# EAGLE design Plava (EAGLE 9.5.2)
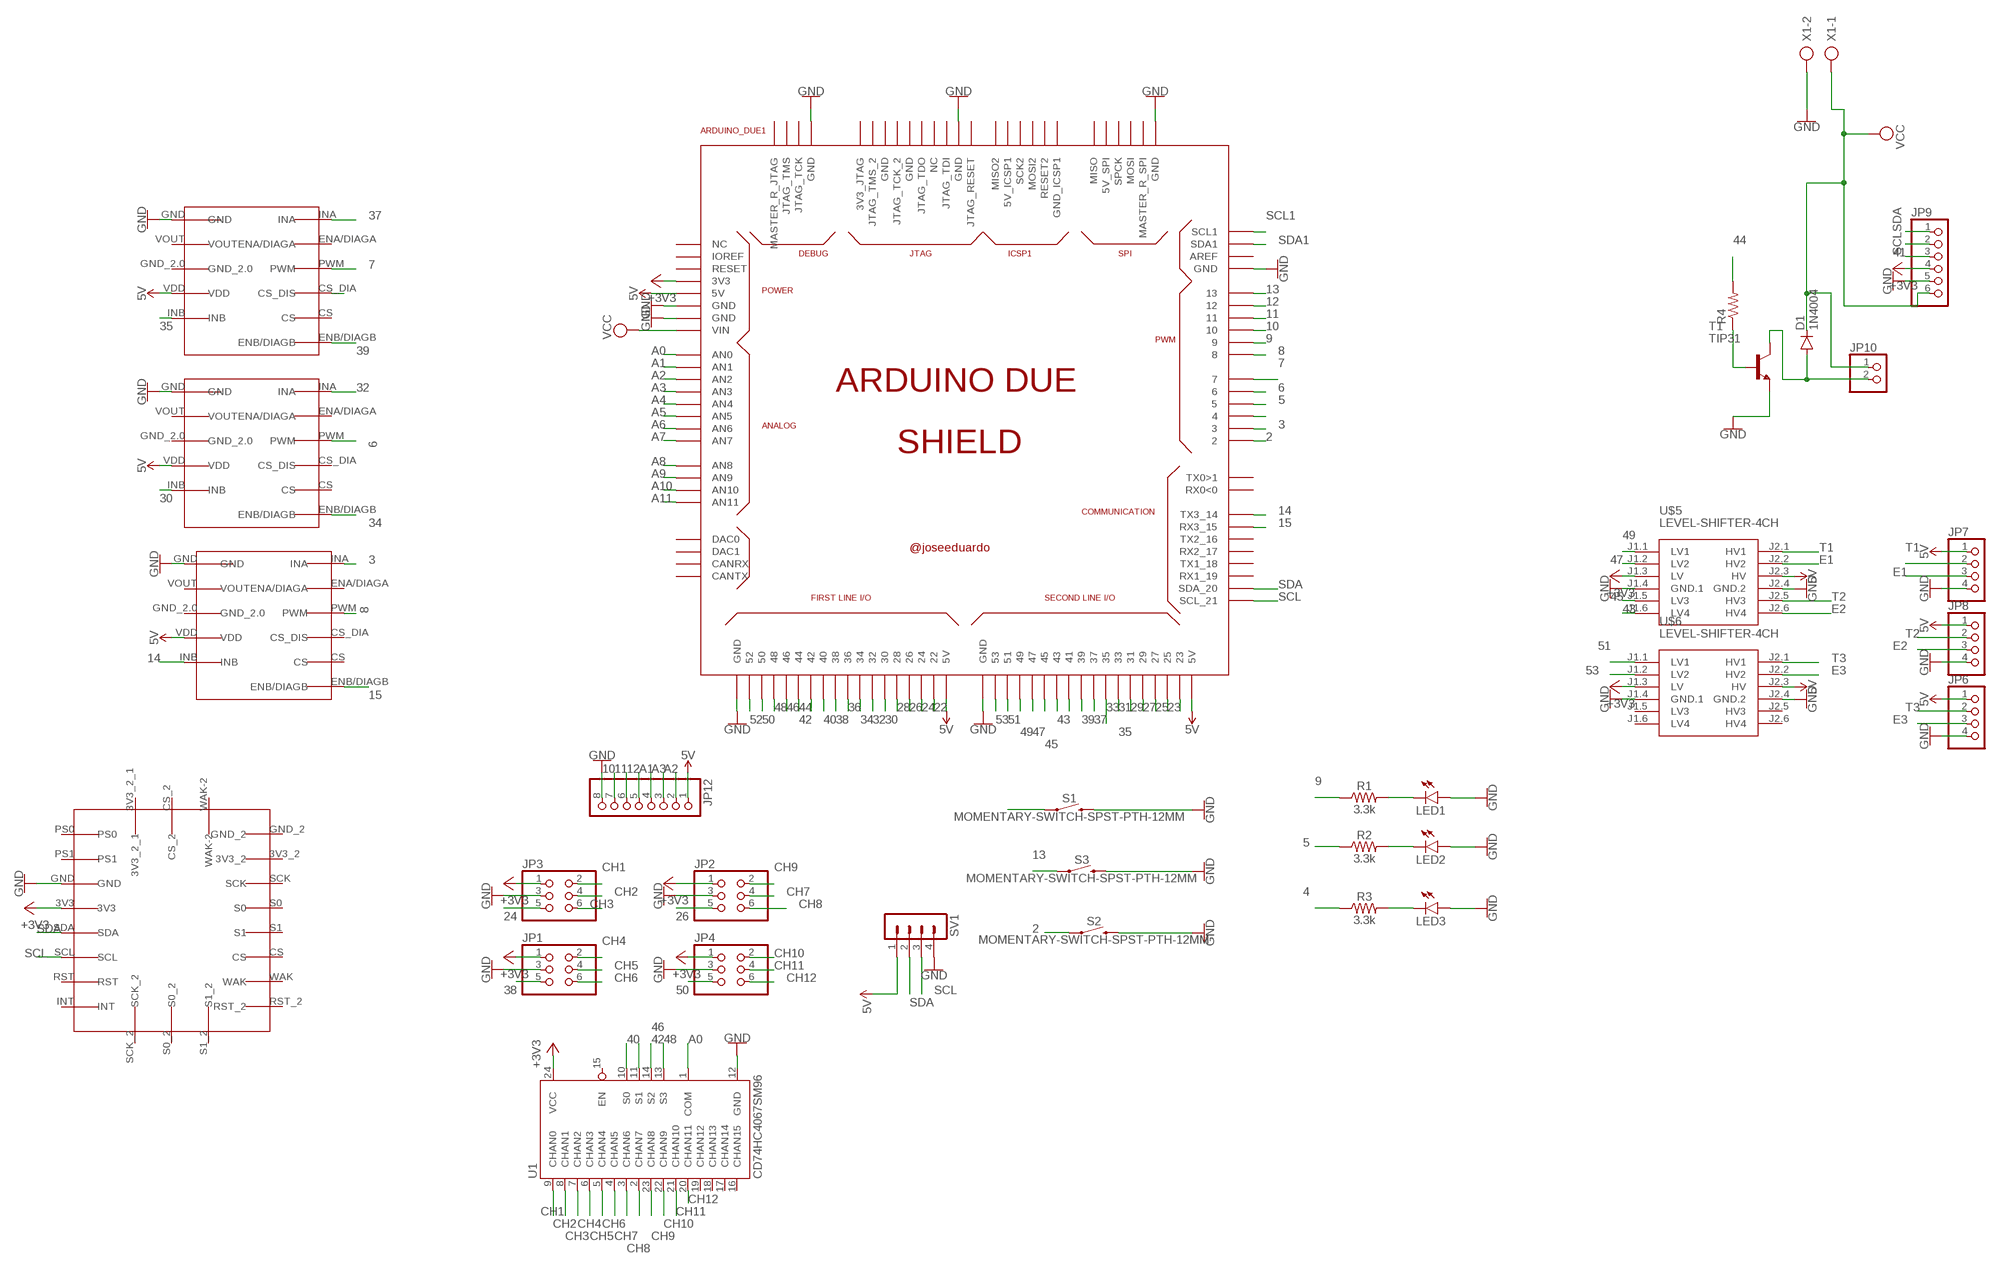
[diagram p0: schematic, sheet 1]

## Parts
ARDUINO_DUE1  ARDUINO_DUE_SHIELD  [ARDUINO_DUE_SHIELD]
D1  1N4004  [DO41-10]
JP1  PINHD-2X3  [2X03]
JP2  PINHD-2X3  [2X03]
JP3  PINHD-2X3  [2X03]
JP4  PINHD-2X3  [2X03]
JP6  PINHD-1X4  [1X04]
JP7  PINHD-1X4  [1X04]
JP8  PINHD-1X4  [1X04]
JP9  PINHD-1X6  [1X06]
JP10  PINHD-1X2  [1X02]
JP12  PINHD-1X8CLEANBIG  [1X08-CLEANBIG]
LED1  LEDCHIP-LED0603  [CHIP-LED0603]
LED2  LEDCHIP-LED0603  [CHIP-LED0603]
LED3  LEDCHIP-LED0603  [CHIP-LED0603]
R1  3.3k  3.3KOHM-0603-1/10W-1%  [0603]
R2  3.3k  3.3KOHM-0603-1/10W-1%  [0603]
R3  3.3k  3.3KOHM-0603-1/10W-1%  [0603]
R4  R-US_0207/7  [0207/7]
S1  MOMENTARY-SWITCH-SPST-PTH-12MM  [TACTILE_SWITCH_PTH_12MM]
S2  MOMENTARY-SWITCH-SPST-PTH-12MM  [TACTILE_SWITCH_PTH_12MM]
S3  MOMENTARY-SWITCH-SPST-PTH-12MM  [TACTILE_SWITCH_PTH_12MM]
SV1  MA04-1  [MA04-1]
T1  TIP31  [TO220]
U1  CD74HC4067SM96  74HC4067SM96  [SSOP24]
U$1  VNH5019_MODULE  [VNH5019]
U$2  VNH5019_MODULE  [VNH5019]
U$3  VNH5019_MODULE  [VNH5019]
U$4  IMU_BNO080  [IMU_BNO080]
U$5  LEVEL-SHIFTER-4CH  [LEVEL-SHIFTER-4CH]
U$6  LEVEL-SHIFTER-4CH  [LEVEL-SHIFTER-4CH]
X1  AK500/2  [AK500/2]

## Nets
2: ARDUINO_DUE1.2 S2.1
3: ARDUINO_DUE1.3 U$3.INA
4: ARDUINO_DUE1.4 R3.1
5: ARDUINO_DUE1.5 R2.1
5V: ARDUINO_DUE1.5V0(5V) ARDUINO_DUE1.5V0_1(5V) ARDUINO_DUE1.5V0_2(5V) JP6.1 JP7.1 JP8.1 JP12.1 SV1.1 U$1.VDD U$2.VDD U$3.VDD U$5.J2.3(HV) U$6.J2.3(HV)
6: ARDUINO_DUE1.6 U$2.PWM
7: ARDUINO_DUE1.7 U$1.PWM
8: ARDUINO_DUE1.8 U$3.PWM
9: ARDUINO_DUE1.9 R1.1
10: ARDUINO_DUE1.10 JP12.7
11: ARDUINO_DUE1.11 JP12.6
12: ARDUINO_DUE1.12 JP12.5
13: ARDUINO_DUE1.13 S3.1
14: ARDUINO_DUE1.14(TX3_14) U$3.INB
15: ARDUINO_DUE1.15(RX3_15) U$3.ENB/DIAGB
22: ARDUINO_DUE1.22
23: ARDUINO_DUE1.23
24: ARDUINO_DUE1.24 JP3.5
25: ARDUINO_DUE1.25
26: ARDUINO_DUE1.26 JP2.5
27: ARDUINO_DUE1.27
28: ARDUINO_DUE1.28
29: ARDUINO_DUE1.29
30: ARDUINO_DUE1.30 U$2.INB
31: ARDUINO_DUE1.31
32: ARDUINO_DUE1.32 U$2.INA
33: ARDUINO_DUE1.33
34: ARDUINO_DUE1.34 U$2.ENB/DIAGB
35: ARDUINO_DUE1.35 U$1.INB
36: ARDUINO_DUE1.36
37: ARDUINO_DUE1.37 U$1.INA
38: ARDUINO_DUE1.38 JP1.5
39: ARDUINO_DUE1.39 U$1.ENB/DIAGB
40: ARDUINO_DUE1.40 U1.10(S0)
41: ARDUINO_DUE1.41 JP9.3
42: ARDUINO_DUE1.42 U1.11(S1)
43: ARDUINO_DUE1.43 U$5.J1.6(LV4)
44: ARDUINO_DUE1.44 R4.2
45: ARDUINO_DUE1.45 U$5.J1.5(LV3)
46: ARDUINO_DUE1.46 U1.14(S2)
47: ARDUINO_DUE1.47 U$5.J1.2(LV2)
48: ARDUINO_DUE1.48 U1.13(S3)
49: ARDUINO_DUE1.49 U$5.J1.1(LV1)
50: ARDUINO_DUE1.50 JP4.5
51: ARDUINO_DUE1.51 U$6.J1.1(LV1)
52: ARDUINO_DUE1.52 S1.1
53: ARDUINO_DUE1.53 U$6.J1.2(LV2)
+3V3: ARDUINO_DUE1.3V3 JP1.1 JP2.1 JP3.1 JP4.1 JP9.4 U1.24(VCC) U$4.3V3 U$5.J1.3(LV) U$6.J1.3(LV)
A0: ARDUINO_DUE1.A0(AN0) U1.1(COM)
A1: ARDUINO_DUE1.A1(AN1) JP12.4
A2: ARDUINO_DUE1.A2(AN2) JP12.2
A3: ARDUINO_DUE1.A3(AN3) JP12.3
A4: ARDUINO_DUE1.A4(AN4)
A5: ARDUINO_DUE1.A5(AN5)
A6: ARDUINO_DUE1.A6(AN6)
A7: ARDUINO_DUE1.A7(AN7)
A8: ARDUINO_DUE1.A8(AN8)
A9: ARDUINO_DUE1.A9(AN9)
A10: ARDUINO_DUE1.A10(AN10)
A11: ARDUINO_DUE1.A11(AN11)
CH1: JP3.2 U1.9(CHAN0)
CH2: JP3.4 U1.8(CHAN1)
CH3: JP3.6 U1.7(CHAN2)
CH4: JP1.2 U1.6(CHAN3)
CH5: JP1.4 U1.5(CHAN4)
CH6: JP1.6 U1.4(CHAN5)
CH7: JP2.4 U1.3(CHAN6)
CH8: JP2.6 U1.2(CHAN7)
CH9: JP2.2 U1.23(CHAN8)
CH10: JP4.2 U1.22(CHAN9)
CH11: JP4.4 U1.21(CHAN10)
CH12: JP4.6 U1.20(CHAN11)
E1: JP7.3 U$5.J2.2(HV2)
E2: JP8.3 U$5.J2.6(HV4)
E3: JP6.3 U$6.J2.2(HV2)
GND: ARDUINO_DUE1.GND ARDUINO_DUE1.GND_1(GND) ARDUINO_DUE1.GND_2(GND) ARDUINO_DUE1.GND_3(GND) ARDUINO_DUE1.GND_4(GND) ARDUINO_DUE1.GND_5(GND) ARDUINO_DUE1.GND_7(GND) ARDUINO_DUE1.GND_10(GND) JP1.3 JP2.3 JP3.3 JP4.3 JP6.4 JP7.4 JP8.4 JP9.5 JP12.8 LED1.A LED2.A LED3.A S1.3 S2.3 S3.3 SV1.4 T1.3(E) U1.12(GND) U$1.GND U$2.GND U$3.GND U$4.GND U$5.J1.4(GND.1) U$5.J2.4(GND.2) U$6.J1.4(GND.1) U$6.J2.4(GND.2) X1.2
N$1: LED1.C R1.2
N$2: LED2.C R2.2
N$3: LED3.C R3.2
N$4: D1.A JP10.2 T1.2(C)
N$5: R4.1 T1.1(B)
N$9: U$1.CS_DIA(CS_DIS)
SCL: ARDUINO_DUE1.21(SCL_21) JP9.2 SV1.3 U$4.SCL
SCL1: ARDUINO_DUE1.SCL1
SDA: ARDUINO_DUE1.20(SDA_20) JP9.1 SV1.2 U$4.SDA
SDA1: ARDUINO_DUE1.SDA1
T1: JP7.2 U$5.J2.1(HV1)
T2: JP8.2 U$5.J2.5(HV3)
T3: JP6.2 U$6.J2.1(HV1)
VCC: ARDUINO_DUE1.VIN D1.C JP9.6 JP10.1 X1.1
Unconnected: ARDUINO_DUE1.0(RX0<0) ARDUINO_DUE1.1(TX0>1) ARDUINO_DUE1.3V3_JTAG ARDUINO_DUE1.5V_2(5V_SPI) ARDUINO_DUE1.5V_ICSP1 ARDUINO_DUE1.16(TX2_16) ARDUINO_DUE1.17(RX2_17) ARDUINO_DUE1.18(TX1_18) ARDUINO_DUE1.19(RX1_19) ARDUINO_DUE1.AREF ARDUINO_DUE1.CANRX ARDUINO_DUE1.CANTX ARDUINO_DUE1.DAC0 ARDUINO_DUE1.DAC1 ARDUINO_DUE1.GND_8(GND) ARDUINO_DUE1.GND_9(GND) ARDUINO_DUE1.GND_ICSP1 ARDUINO_DUE1.IOREF ARDUINO_DUE1.JTAG_RESET ARDUINO_DUE1.JTAG_TCK ARDUINO_DUE1.JTAG_TCK_2 ARDUINO_DUE1.JTAG_TDI ARDUINO_DUE1.JTAG_TDO ARDUINO_DUE1.JTAG_TMS ARDUINO_DUE1.JTAG_TMS_2 ARDUINO_DUE1.MASTER_RESET_JTAG(MASTER_R_JTAG) ARDUINO_DUE1.MASTER_RESET_SPI(MASTER_R_SPI) ARDUINO_DUE1.MISO ARDUINO_DUE1.MISO2 ARDUINO_DUE1.MOSI ARDUINO_DUE1.MOSI2 ARDUINO_DUE1.NC_2(NC) ARDUINO_DUE1.NC_5(NC) ARDUINO_DUE1.RESET ARDUINO_DUE1.RESET2 ARDUINO_DUE1.SCK2 ARDUINO_DUE1.SPCK U1.15(EN) U1.16(CHAN15) U1.17(CHAN14) U1.18(CHAN13) U1.19(CHAN12) U$1.CS U$1.ENA/DIAGA U$1.GND_2.0 U$1.VOUT U$2.CS U$2.CS_DIA(CS_DIS) U$2.ENA/DIAGA U$2.GND_2.0 U$2.VOUT U$3.CS U$3.CS_DIA(CS_DIS) U$3.ENA/DIAGA U$3.GND_2.0 U$3.VOUT U$4.3V3_2 U$4.3V3_2_1 U$4.CS U$4.CS_2 U$4.GND_2 U$4.INT U$4.PS0 U$4.PS1 U$4.RST U$4.RST_2 U$4.S0 U$4.S0_2 U$4.S1 U$4.S1_2 U$4.SCK U$4.SCK_2 U$4.WAK U$4.WAK-2 U$6.J1.5(LV3) U$6.J1.6(LV4) U$6.J2.5(HV3) U$6.J2.6(HV4)

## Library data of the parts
ARDUINO_DUE1 = arduino_due_shield:ARDUINO_DUE_SHIELD
D1 = diode:1N4004: DIODE
JP1-JP4 = pinhead:PINHD-2X3: PIN HEADER
JP6-JP8 = pinhead:PINHD-1X4: PIN HEADER
JP9 = adafruit:PINHD-1X6: PIN HEADER
JP10 = pinhead:PINHD-1X2: PIN HEADER
JP12 = adafruit:PINHD-1X8: PIN HEADER
LED1-LED3 = led:LED: LED
R1-R3 = SparkFun-Resistors:3.3KOHM: 3.3kΩ resistor; PROD_ID: RES-07851
R4 = rcl:R-US_: RESISTOR, American symbol; SPICEPREFIX: R
S1-S3 = SparkFun-Switches:MOMENTARY-SWITCH-SPST: Momentary Switch (Pushbutton) - SPST; PROD_ID: SWCH-09185; SF_SKU: COM-09190
SV1 = con-lstb:MA04-1: PIN HEADER; OC_FARNELL: unknown; OC_NEWARK: unknown
T1 = transistor:TIP31: NPN Transistor Medium Power Linear Switching Applications Source: http://onsemi.com
U1 = SparkFun-IC-Logic:74*4067: 16-channel analog MUX Datasheet SparkFun Products MP3 Trigger (WIG-13720) SparkFun Analog/Digital MUX Breakout - CD74HC4067 (BOB-09056); PROD_ID: IC-08252
U$1-U$3 = Puente_h_mamalon:VNH5019_MODULE
U$4 = IMU bno080:IMU_BNO080
U$5 U$6 = diy-modules:LEVEL-SHIFTER-4CH: 4-Channel Bi-Directional Logic Level Converter based on BSS128 transistors Click here to find device on ebay.com
X1 = con-ptr500:AK500/2: CONNECTOR; OC_FARNELL: unknown; OC_NEWARK: unknown

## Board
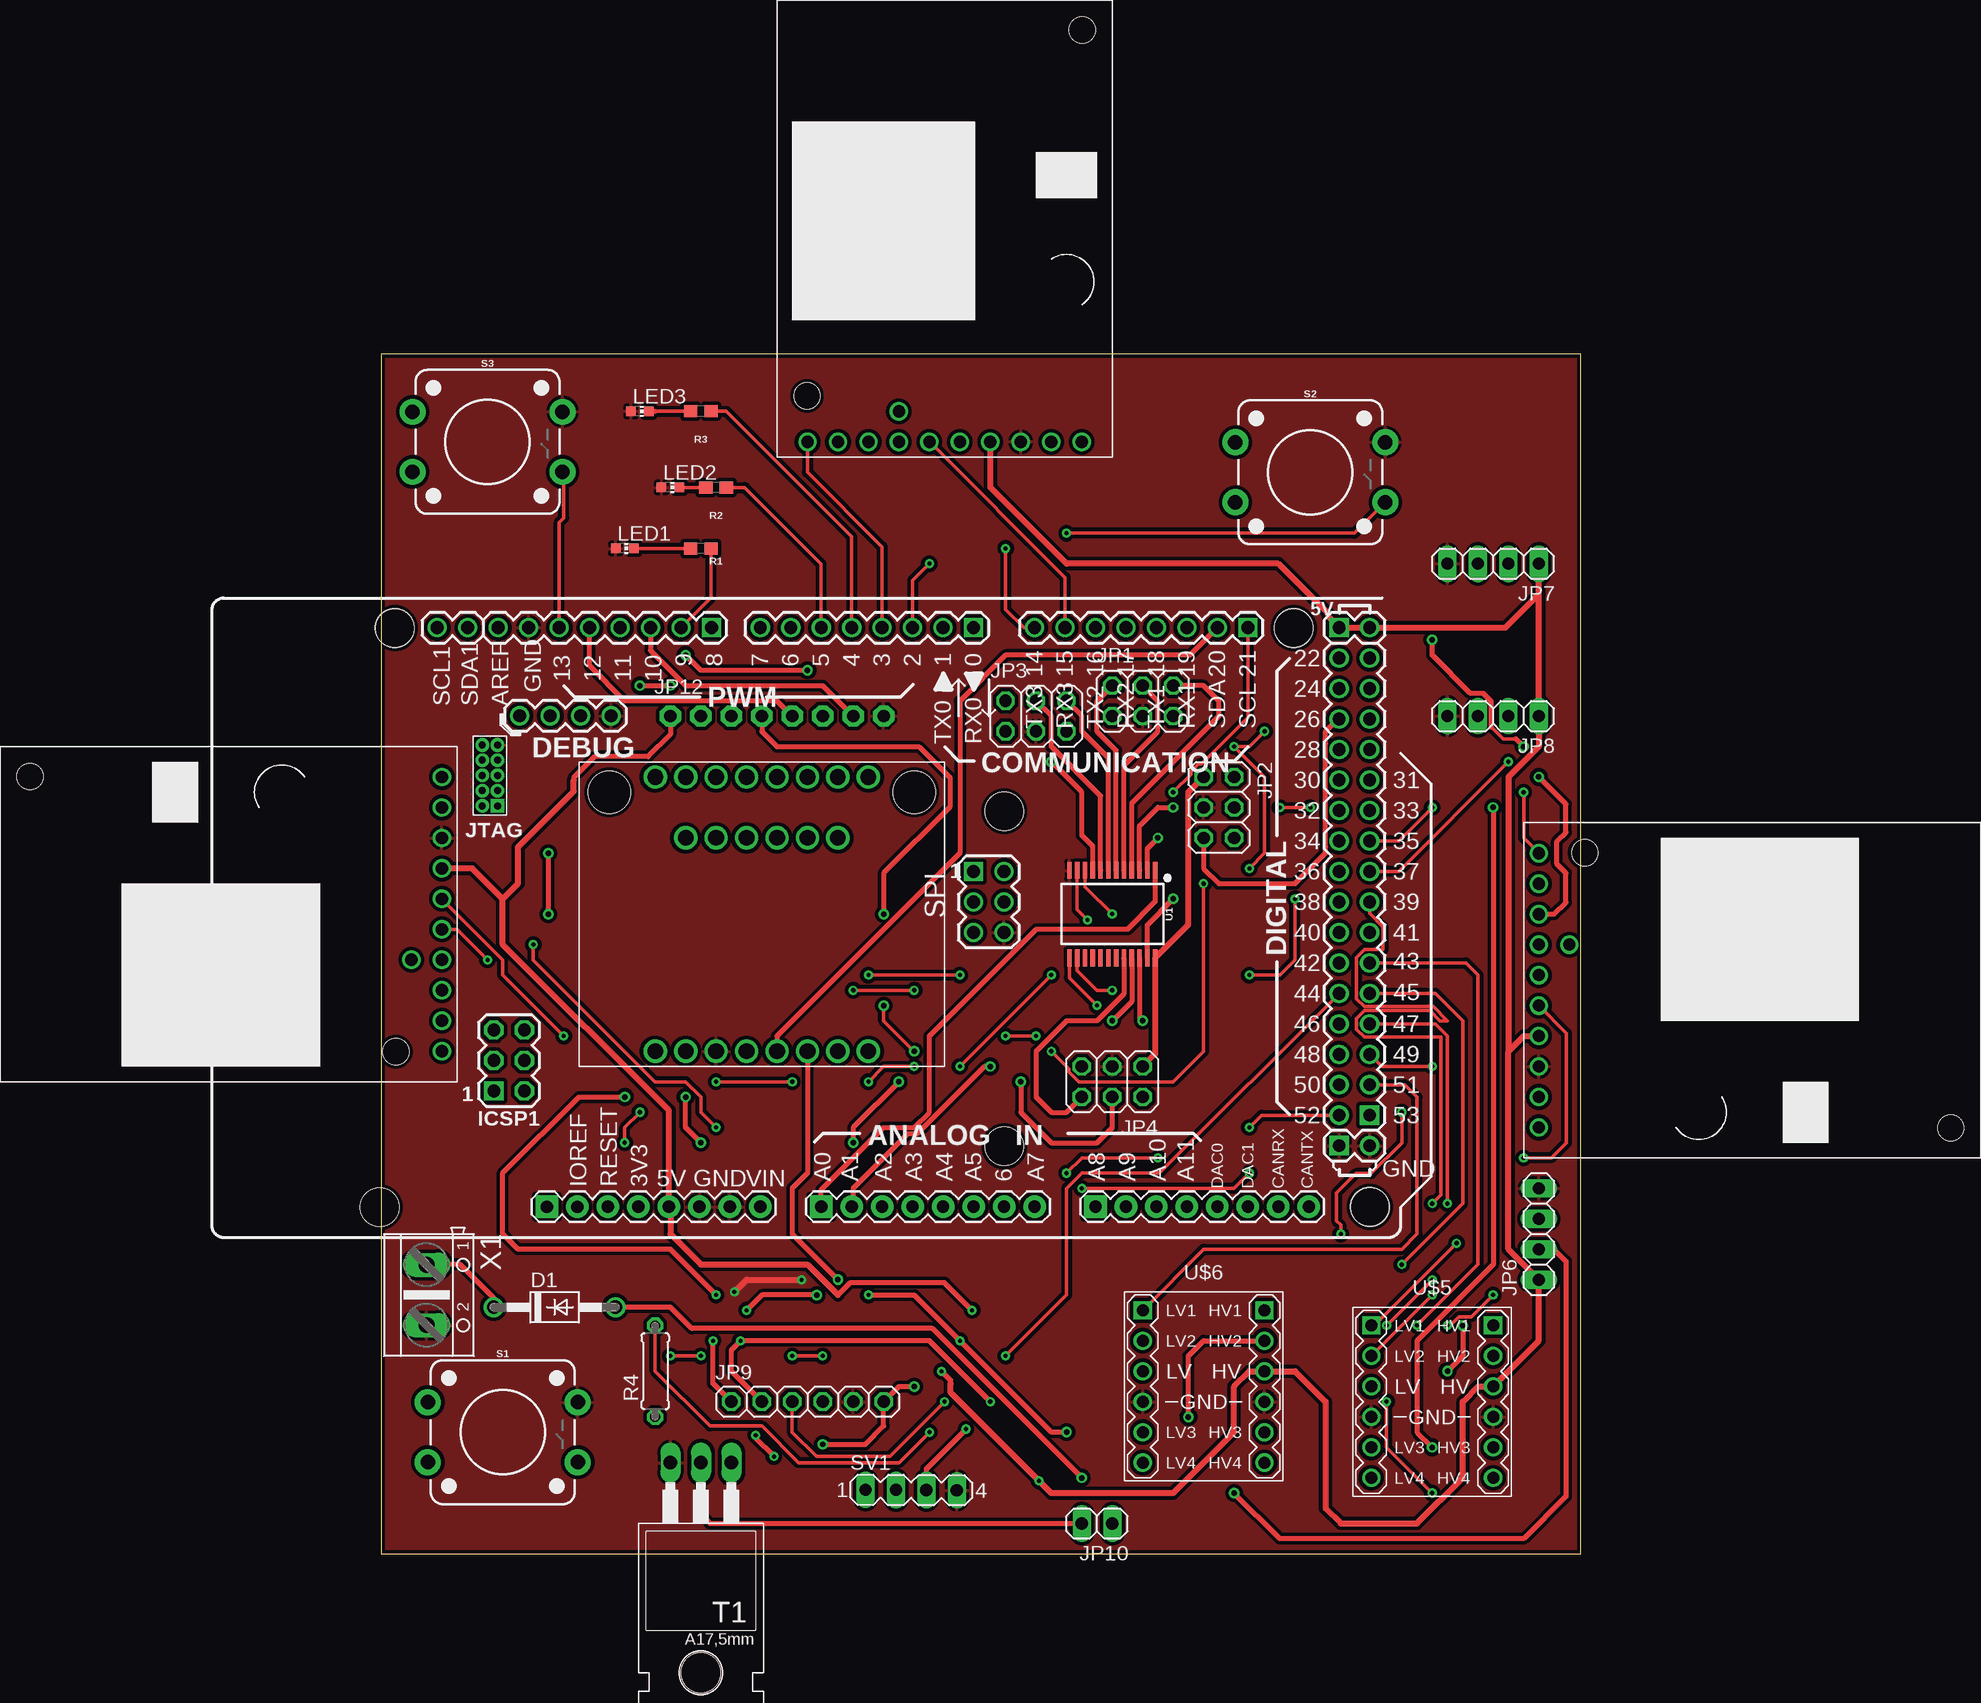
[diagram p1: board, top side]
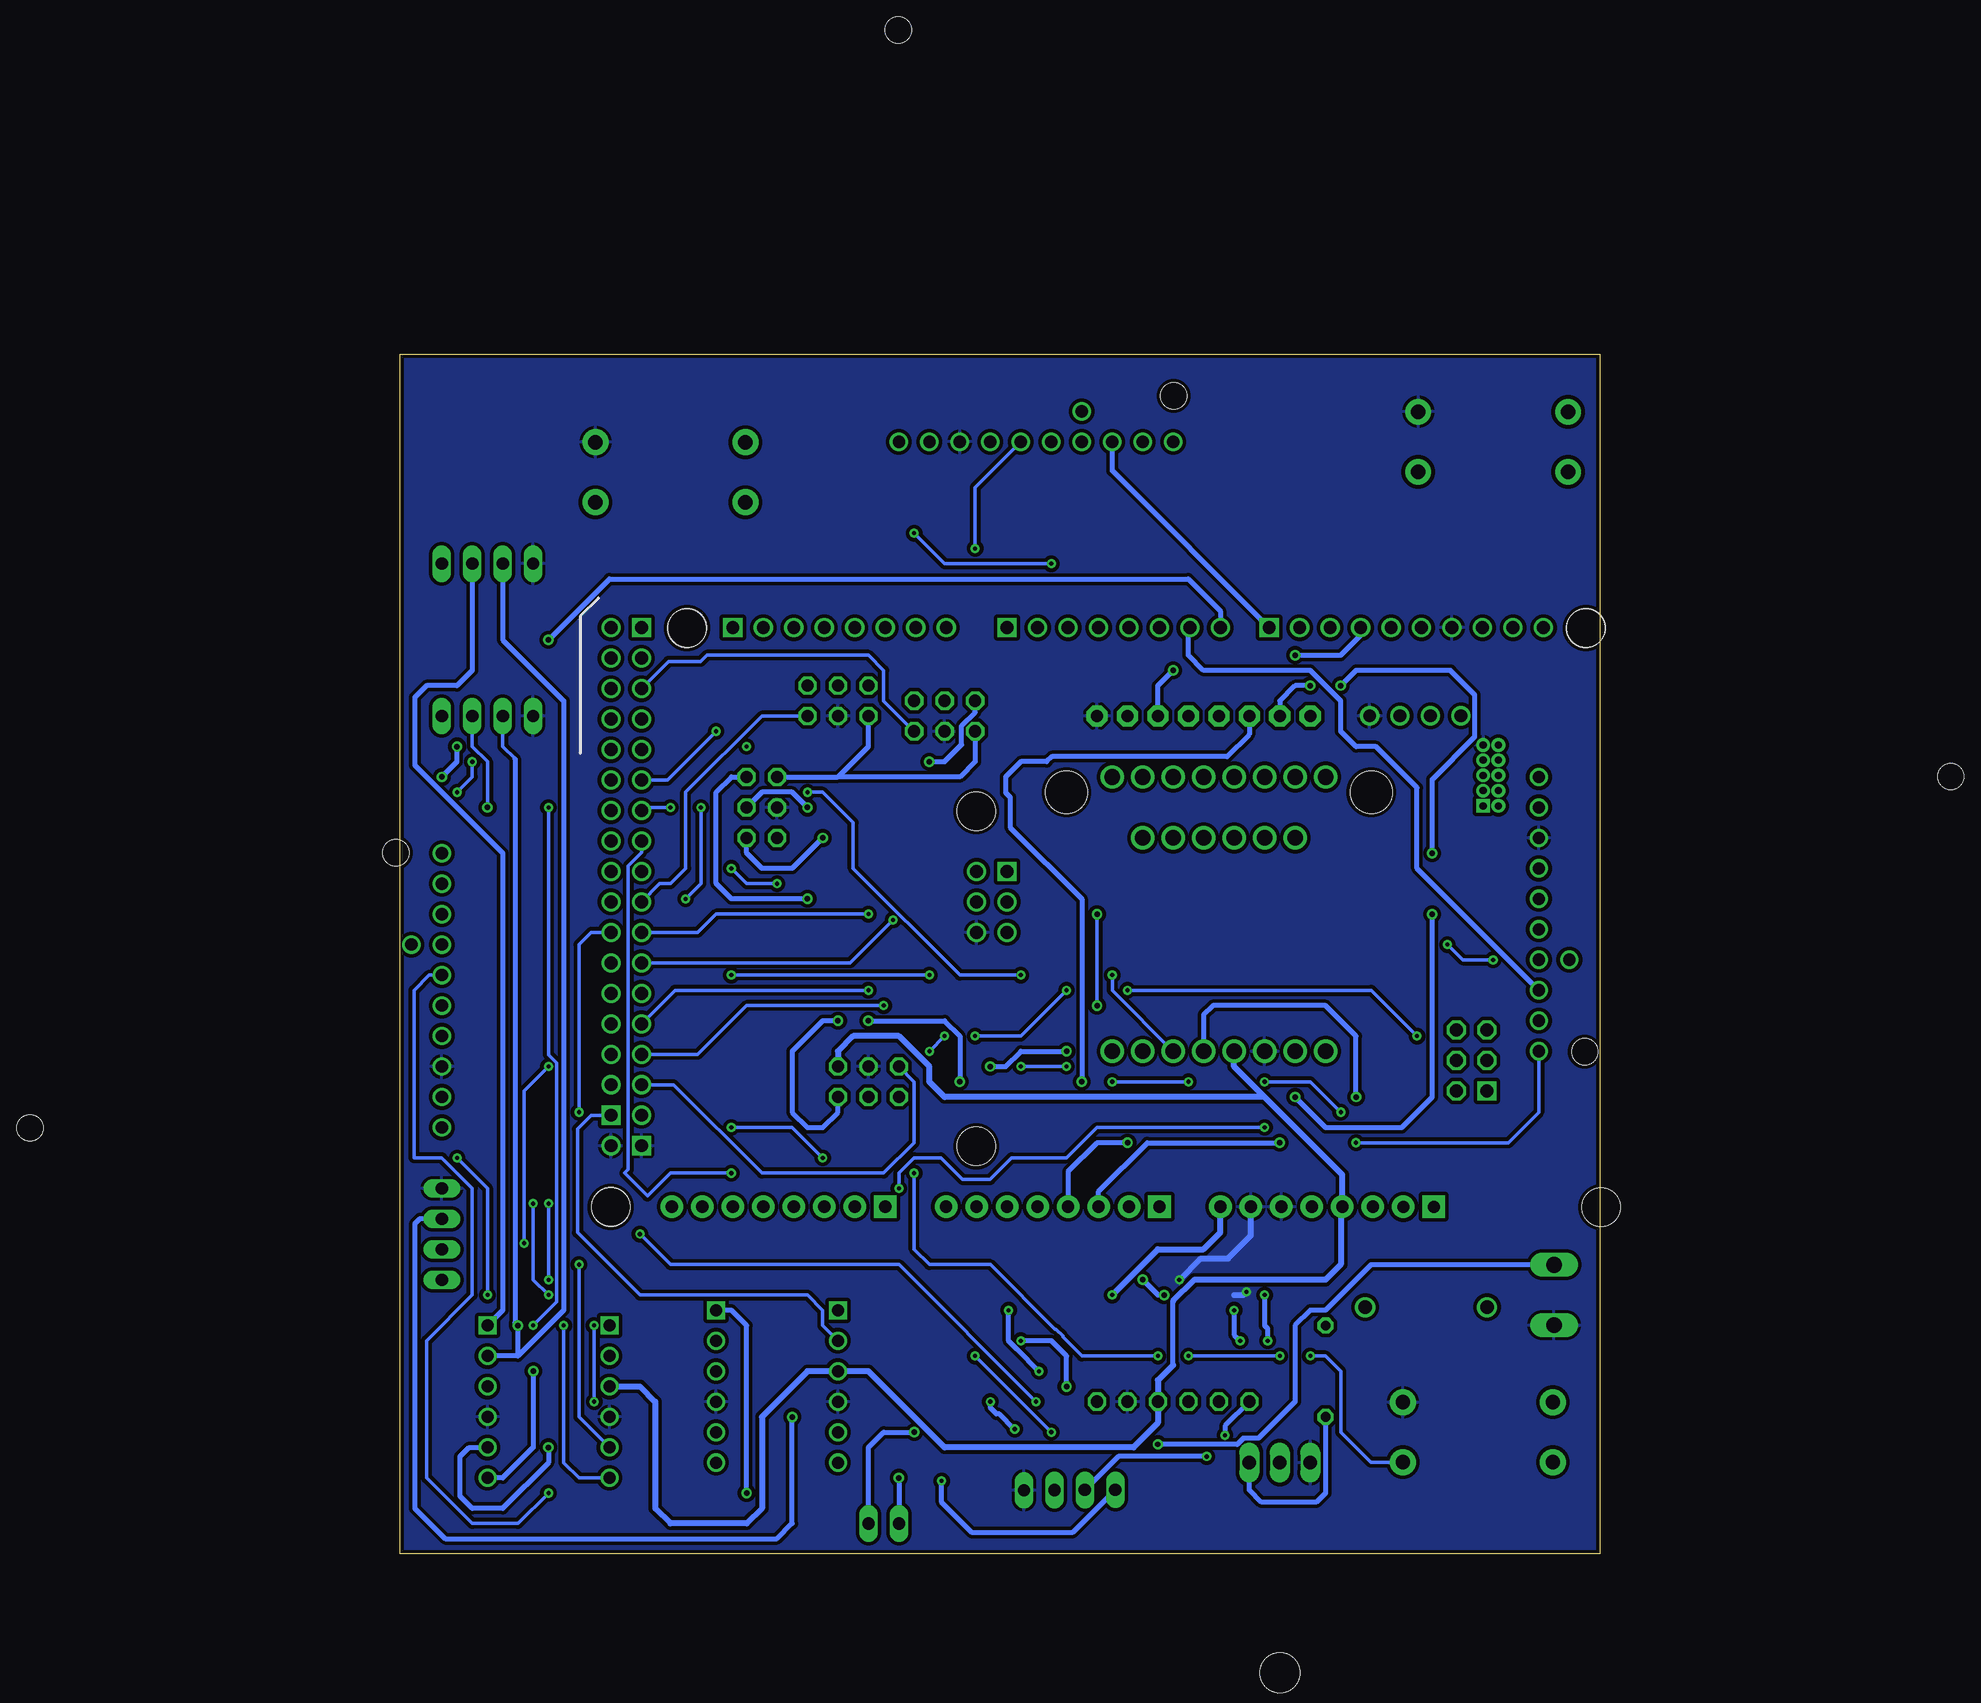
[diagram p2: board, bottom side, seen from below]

Size 100 x 100 mm. Coordinates in mm from the lower left corner, seen from the top.
Outline: 0,0 100,0 100,100 0,100 0,0
Copper layers (1*16): Top 0.035mm / dielectric 1.5mm / Bottom 0.035mm
Design rules "default *": minimum track width 6mil, minimum drill 0.35mm, track to track 6mil, track to pad 6mil, pad to pad 6mil, via to via 6mil, smd to smd 6mil, copper to edge 10mil, drill to drill 6mil, minimum pad ring 10mil, minimum via ring 8mil, stop-mask expansion 4mil, vias tented up to drill 0mil, thermal gap 10mil

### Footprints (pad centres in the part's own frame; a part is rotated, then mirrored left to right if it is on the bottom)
ARDUINO_DUE_SHIELD = drill 1.067 square: 0 63.373,51.816; 5V0_1 93.853,51.816; 8 41.529,51.816; 21 86.233,51.816; 53 96.393,11.176; GND_2 93.853,8.636; MISO 63.373,31.496; MISO2 23.384,13.196 | drill 1.067: 1 60.833,51.816; 2 58.293,51.816; 3 55.753,51.816; 4 53.213,51.816; 5 50.673,51.816; 5V0_2 96.393,51.816; 5V_2 65.913,31.496; 6 48.133,51.816; 7 45.593,51.816; 9 38.989,51.816; 10 36.449,51.816; 11 33.909,51.816; 12 31.369,51.816; 13 28.829,51.816; 14 68.453,51.816; 15 70.993,51.816; 16 73.533,51.816; 17 76.073,51.816; 18 78.613,51.816; 19 81.153,51.816; 20 83.693,51.816; 22 93.853,49.276; 23 96.393,49.276; 24 93.853,46.736; 25 96.393,46.736; 26 93.853,44.196; 27 96.393,44.196; 28 93.853,41.656; 29 96.393,41.656; 30 93.853,39.116; 31 96.393,39.116; 32 93.853,36.576; 33 96.393,36.576; 34 93.853,34.036; 35 96.393,34.036; 36 93.853,31.496; 37 96.393,31.496; 38 93.853,28.956; 39 96.393,28.956; 40 93.853,26.416; 41 96.393,26.416; 42 93.853,23.876; 43 96.393,23.876; 44 93.853,21.336; 45 96.393,21.336; 46 93.853,18.796; 47 96.393,18.796; 48 93.853,16.256; 49 96.393,16.256; 50 93.853,13.716; 51 96.393,13.716; 52 93.853,11.176; AREF 23.749,51.816; GND_3 96.393,8.636; GND_4 26.289,51.816; GND_5 65.913,26.416; GND_7 33.161,44.473; JTAG_TCK 30.621,44.473; JTAG_TMS 28.081,44.473; MASTER_RESET_JTAG 25.541,44.473; MASTER_RESET_SPI 63.373,26.416; MOSI 65.913,28.956; SCL1 18.669,51.816; SDA1 21.209,51.816; SPCK 63.373,28.956 | drill 1.016 pad 1.88: 3V3 35.433,3.556; 5V0 37.973,3.556; A1 53.213,3.556; A2 55.753,3.556; A3 58.293,3.556; A4 60.833,3.556; A5 63.373,3.556; A6 65.913,3.556; A7 68.453,3.556; A9 76.073,3.556; A10 78.613,3.556; A11 81.153,3.556; CANRX 88.773,3.556; CANTX 91.313,3.556; DAC0 83.693,3.556; DAC1 86.233,3.556; GND 40.513,3.556; GND_1 43.053,3.556; IOREF 30.346,3.543; RESET 32.893,3.555; VIN 45.593,3.556 | drill 0.6 pad 1.016 square: 3V3_JTAG 23.689,36.964 | drill 1.067 octagon: 5V_ICSP1 25.924,13.196; GND_ICSP1 25.924,18.276; MOSI2 25.924,15.736; RESET2 23.384,18.276; SCK2 23.384,15.736 | drill 1.016 pad 1.88 square: A0 50.673,3.556; A8 73.533,3.556; NC_2 27.806,3.543 | drill 0.6 pad 1.143: GND_8 23.689,38.234; GND_9 23.689,40.774; GND_10 23.689,42.044; JTAG_RESET 22.419,42.044; JTAG_TCK_2 22.419,38.234; JTAG_TDI 22.419,40.774; JTAG_TDO 22.419,39.504; JTAG_TMS_2 22.419,36.964; NC_5 23.689,39.504 | hole 3.2: 15.113,51.816; 90.043,51.816; 96.393,3.556; 96.418,3.505; 15.138,51.765; 90.068,51.765; 13.868,3.505; 65.938,36.525; 65.938,8.585
DO41-10 = drill 1.118: A 5.08,0; C -5.08,0
2X03 = drill 1.016 octagon: 1 -2.54,-1.27; 2 -2.54,1.27; 3 0,-1.27; 4 0,1.27; 5 2.54,-1.27; 6 2.54,1.27
1X04 = drill 1.016 long: 1 -3.81,0; 2 -1.27,0; 3 1.27,0; 4 3.81,0
1X06 = drill 1.016 octagon: 1 -6.35,0; 2 -3.81,0; 3 -1.27,0; 4 1.27,0; 5 3.81,0; 6 6.35,0
1X02 = drill 1.016 long: 1 -1.27,0; 2 1.27,0
1X08-CLEANBIG = drill 1.016 pad 1.778 octagon: 1 -8.89,0; 2 -6.35,0; 3 -3.81,0; 4 -1.27,0; 5 1.27,0; 6 3.81,0; 7 6.35,0; 8 8.89,0
CHIP-LED0603 = smd 0.8 x 0.8: A 0,-0.75; C 0,0.75
0603 = smd 1.1 x 1: 1 -0.85,0; 2 0.85,0
0207/7 = drill 0.813 octagon: 1 -3.81,0; 2 3.81,0
TACTILE_SWITCH_PTH_12MM = drill 1.2 pad 2.159: 1 6.25,-2.5; 2 -6.25,-2.5; 3 6.25,2.5; 4 -6.25,2.5
MA04-1 = drill 1.016 long: 1 -3.81,0; 2 -1.27,0; 3 1.27,0; 4 3.81,0
TO220 = drill 1.118 long: 1 -2.54,-6.35; 2 0,-6.35; 3 2.54,-6.35 | hole 3.302: 0,11.176
SSOP24 = smd 0.348 x 1.397: 1 -3.575,-3.656; 2 -2.925,-3.656; 3 -2.275,-3.656; 4 -1.625,-3.656; 5 -0.975,-3.656; 6 -0.325,-3.656; 7 0.325,-3.656; 8 0.975,-3.656; 9 1.625,-3.656; 10 2.275,-3.656; 11 2.925,-3.656; 12 3.575,-3.656; 13 3.575,3.656; 14 2.925,3.656; 15 2.275,3.656; 16 1.625,3.656; 17 0.975,3.656; 18 0.325,3.656; 19 -0.325,3.656; 20 -0.975,3.656; 21 -1.625,3.656; 22 -2.275,3.656; 23 -2.925,3.656; 24 -3.575,3.656
VNH5019 = drill 1.02: CS 10.16,1.27; CS_DIA 10.16,3.81; ENA/DIAGA 5.08,1.27; ENB/DIAGB 12.7,1.27; GND 20.32,1.27; GND_2.0 25.4,1.27; INA 2.54,1.27; INB 15.24,1.27; PWM 7.62,1.27; VDD 17.78,1.27; VOUT 22.86,1.27 | hole 2.18: 2.5,5.1; 25.44,35.6
IMU_BNO080 = drill 1.3: 3V3 13.97,1.27; 3V3_2 8.89,24.13; 3V3_2_1 8.89,19.05; CS 19.05,24.13; CS_2 19.05,19.05; GND 11.43,1.27; GND_2 6.35,24.13; INT 24.13,1.27; PS0 6.35,1.27; PS1 8.89,1.27; RST 21.59,1.27; RST_2 24.13,24.13; S0 13.97,24.13; S0_2 13.97,19.05; S1 16.51,24.13; S1_2 16.51,19.05; SCK 11.43,24.13; SCK_2 11.43,19.05; SCL 19.05,1.27; SDA 16.51,1.27; WAK 21.59,24.13; WAK-2 21.59,19.05 | hole 3.5: 2.54,22.86; 27.94,22.86
LEVEL-SHIFTER-4CH = drill 1 square: J1.1 -5.08,6.35; J2.1 5.08,6.35 | drill 1: J1.2 -5.08,3.81; J1.3 -5.08,1.27; J1.4 -5.08,-1.27; J1.5 -5.08,-3.81; J1.6 -5.08,-6.35; J2.2 5.08,3.81; J2.3 5.08,1.27; J2.4 5.08,-1.27; J2.5 5.08,-3.81; J2.6 5.08,-6.35
AK500/2 = drill 1.321 long: 1 -2.515,0; 2 2.515,0

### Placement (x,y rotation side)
ARDUINO_DUE1  -13.97,25.4 0 top
D1  14.48,20.57 0 top
JP1  63.5,71.12 0 top
JP2  69.85,62.23 270 top
JP3  54.61,69.85 0 top
JP4  60.96,39.37 180 top
JP6  96.52,26.67 90 top
JP7  92.71,82.55 180 top
JP8  92.71,69.85 180 top
JP9  35.56,12.7 0 top
JP10  59.69,2.54 180 top
JP12  33.02,69.85 0 top
LED1  20.32,83.82 270 top
LED2  24.13,88.9 270 top
LED3  21.59,95.25 270 top
R1  26.67,83.82 180 top
R2  27.94,88.9 180 top
R3  26.67,95.25 180 top
R4  22.86,15.24 90 top
S1  10.16,10.16 0 top
S2  77.47,90.17 0 top
S3  8.89,92.71 0 top
SV1  44.2,5.33 359.7 top
T1  26.67,1.27 180 top
U1  60.96,53.34 180 top
U$1  95.25,60.96 270 top
U$2  6.35,39.37 90 top
U$3  33.02,91.44 0 top
U$4  16.51,40.64 0 top
U$5  87.63,12.7 0 top
U$6  68.58,13.97 0 top
X1  3.81,21.59 270 top

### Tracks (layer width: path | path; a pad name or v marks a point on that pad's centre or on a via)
2  (via drill 0.35)
  Top 0.305: S2.1 81.14,85.09 v57.15,85.09 | v45.72,82.55 44.32,81.15 ARDUINO_DUE1.2
  Bottom 0.305: v57.15,85.09 54.61,82.55 v45.72,82.55
3
  Top 0.305: U$3.INA 35.56,90.17 41.78,83.95 ARDUINO_DUE1.3
4
  Top 0.305: R3.1 28.79,95.25 39.24,84.8 ARDUINO_DUE1.4
5
  Top 0.305: R2.1 30.31,88.9 36.7,82.51 ARDUINO_DUE1.5
5V  (via drill 0.35)
  Top 0.406: JP12.1 24.13,68.33 22.27,66.47 17.82,66.47 16.08,64.73 16.08,64.52 | 47.5,14.22 47.5,14.48 v46.74,15.24 | v49.28,20.32 46.99,22.61 39.12,22.61 38.1,21.59
  Top 0.508: 38.1,21.59 35.56,24.13 26.67,24.13 24.13,26.67 24.13,28.83 ARDUINO_DUE1.5V0 24,36.96 10.16,50.8 10.16,54.61 | 96.52,80.01 93.73,77.22 ARDUINO_DUE1.5V0_2 ARDUINO_DUE1.5V0_1 78.97,78.13 78.97,78.38 74.8,82.55 57.15,82.55 50.8,88.9 U$3.VDD | 96.52,80.01 JP7.1 | 96.52,80.01 JP8.1 96.52,67.31 93.98,64.77 93.98,41.91 | 10.16,54.61 7.62,57.15 U$2.VDD | 93.98,41.91 95.25,43.18 U$1.VDD | 93.98,41.91 93.98,25.4 JP6.1 96.52,17.78 U$5.J2.3 91.44,13.97 90.17,12.7 90.17,6.35 86.36,2.54 80.01,2.54 78.74,3.81 78.74,12.7 76.2,15.24 U$6.J2.3 72.39,15.24 71.12,13.97 71.12,10.16 66.04,5.08 55.88,5.08 v54.86,6.1 47.5,13.46 47.5,14.22 | 10.16,54.61 11.43,55.88 11.43,58.93 16.08,63.58 16.08,64.52
  Bottom 0.406: SV1.1 43.96,1.78 52.32,1.78 54.86,4.32 v54.86,6.1 | v46.74,15.24 48.54,17.05 48.56,17.05 49.28,17.76 v49.28,20.32
6
  Bottom 0.406: U$2.PWM 15.24,57.15 15.24,63.89 18.66,67.31 20.32,67.31 21.59,68.58 21.59,71.12 24.13,73.66 33.02,73.66 34.29,74.93 34.29,77.09 ARDUINO_DUE1.6
7  (via drill 0.46)
  Top 0.305: 94.61,67.94 93.54,67.94 92.56,68.93
  Top 0.406: U$1.PWM 97.79,53.34 98.78,54.33 98.78,56.76 98.04,57.5 98.04,59.42 98.78,60.16 98.78,62.51 v96.52,64.77 | v87.63,76.2 87.63,74.93 90.83,71.73 91.9,71.73 92.56,71.08 92.56,68.93 | v95.25,67.31 94.61,67.94 94.59,67.97
  Bottom 0.406: v96.52,64.77 95.25,66.04 v95.25,67.31 | v87.63,76.2 82.55,81.28 34.29,81.28 31.62,78.61 ARDUINO_DUE1.7
8
  Bottom 0.406: ARDUINO_DUE1.8 40.64,90.3 U$3.PWM
9
  Top 0.305: ARDUINO_DUE1.9 27.52,79.72 R1.1
10
  Top 0.406: ARDUINO_DUE1.10 22.48,75.31 25.4,72.39 36.83,72.39 JP12.7
11  (via drill 0.46)
  Top 0.406: v35.56,73.66 26.67,73.66 v25.4,74.93
  Bottom 0.406: JP12.6 36.83,72.39 v35.56,73.66 | v25.4,74.93 21.59,74.93 19.94,76.58 ARDUINO_DUE1.11
12
  Top 0.406: JP12.5 33.02,71.12 20.32,71.12 17.4,74.04 ARDUINO_DUE1.12
13
  Top 0.305: ARDUINO_DUE1.13 14.86,85.98 15.24,86.36 15.24,90.11 S3.1
14  (via drill 0.35)
  Top 0.305: v52.07,83.82 52.07,78.74 53.59,77.22 ARDUINO_DUE1.14
  Bottom 0.305: U$3.INB 52.07,88.9 v52.07,83.82
15
  Top 0.305: U$3.ENB/DIAGB 57.02,81.41 ARDUINO_DUE1.15
24
  Bottom 0.305: ARDUINO_DUE1.24 77.62,74.4 74.95,74.4 74.42,74.93 60.96,74.93 59.69,73.66 59.69,71.12 JP3.5
26
  Top 0.406: JP2.5 68.58,57.15 69.85,55.88 76.2,55.88 78.74,58.42 78.74,58.95 78.73,58.96 78.73,67.53 78.74,67.55 78.74,68.58 79.76,69.6 ARDUINO_DUE1.26
30  (via drill 0.35)
  Top 0.305: v73.66,68.58 72.39,67.31 v71.12,67.31 73.66,64.77 73.66,58.42 v72.39,57.15 | v68.58,55.88 68.58,41.91 66.04,39.37 58.18,39.37 57.35,40.2 57.35,40.44 v55.88,41.91 | v54.61,43.18 v52.07,43.18 | v44.45,46.99 v39.37,46.99 | v15.24,43.18 10.16,48.26 10.16,49.53 U$2.INB
  Bottom 0.305: ARDUINO_DUE1.30 77.72,64.52 v73.66,68.58 | v72.39,57.15 71.12,55.88 v68.58,55.88 | v55.88,41.91 v54.61,43.18 | v52.07,43.18 48.26,43.18 v44.45,46.99 | v39.37,46.99 19.05,46.99 v15.24,43.18
32  (via drill 0.35)
  Top 0.305: v20.32,34.29 20.32,35.56 v21.59,36.83 | v27.94,39.37 v34.29,39.37 | v40.64,39.37 41.91,40.64 v44.45,40.64 | v48.26,40.64 v55.88,48.26 | v72.39,48.26 74.93,48.26 76.2,49.53 v76.2,54.61 | v74.93,62.23 v77.47,62.23
  Bottom 0.305: U$2.INA 5.08,36.83 7.62,34.29 v20.32,34.29 | v21.59,36.83 24.13,39.37 v27.94,39.37 | v34.29,39.37 v40.64,39.37 | v44.45,40.64 v48.26,40.64 | v55.88,48.26 v72.39,48.26 | v76.2,54.61 74.93,55.88 v74.93,62.23 | v77.47,62.23 79.63,62.23 ARDUINO_DUE1.32
34  (via drill 0.35)
  Top 0.305: v72.39,31.75 71.12,30.48 v58.42,30.48 | v27.94,35.56 26.67,36.83 26.67,38.1 25.4,39.37 22.86,39.37 12.7,49.53 v12.7,50.8 | v8.89,49.53 6.35,52.07 U$2.ENB/DIAGB
  Bottom 0.305: ARDUINO_DUE1.34 79.88,58.46 80.99,57.35 80.99,32.04 81.28,31.75 79.38,29.84 77.47,31.75 v72.39,31.75 | v58.42,30.48 58.42,31.75 57.15,33.02 54.92,33.02 53.12,31.22 50.82,31.22 49.02,33.02 44.45,33.02 41.91,35.56 v27.94,35.56 | v12.7,50.8 11.43,49.53 v8.89,49.53
35  (via drill 0.35)
  Top 0.305: U$1.INB 98.83,43.41 98.83,34.29 97.56,33.02 v95.25,33.02 | v92.71,21.59 90.91,19.79 89.86,19.79 89.13,19.05 v88.9,19.05 | v87.63,62.23 84.84,59.44 ARDUINO_DUE1.35
  Bottom 0.305: v95.25,33.02 92.71,30.48 v92.71,21.59 | v87.63,62.23 87.63,41.61 86.95,40.92 86.95,21 v88.9,19.05
37  (via drill 0.35)
  Top 0.305: U$1.INA 95.25,59.69 v95.25,63.5 | v93.98,66.04 84.84,56.9 ARDUINO_DUE1.37
  Bottom 0.305: v95.25,63.5 93.98,64.77 v93.98,66.04
38
  Bottom 0.305: JP1.5 69.85,69.85 76.2,63.5 76.2,57.15 77.47,55.88 78.36,55.88 ARDUINO_DUE1.38
39  (via drill 0.35)
  Top 0.305: ARDUINO_DUE1.39 82.42,53.38 83.53,52.27 83.53,50.38 81.97,50.38 81.32,49.73 81.32,46.28 81.97,45.63 87.72,45.63 88.9,44.45 88.28,44.45 87.43,45.3 81.97,45.3 81.32,44.65 81.32,43.74 81.97,43.09 88.34,43.09 88.34,29.92 v87.63,29.21 | v87.63,22.86 83.83,19.07 v83.83,19.05 | v83.82,12.7 83.82,8.89 v87.63,5.08
  Bottom 0.305: v87.63,29.21 v87.63,22.86 | v83.83,19.05 83.83,12.71 v83.82,12.7 | v87.63,5.08 90.17,2.54 93.98,2.54 97.79,6.35 97.79,17.78 93.98,21.59 93.98,30.48 96.52,33.02 98.83,33.02 98.83,46.99 97.56,48.26 U$1.ENB/DIAGB
40  (via drill 0.35)
  Top 0.305: U1.10 58.69,55.62 v60.96,53.34
  Bottom 0.305: v60.96,53.34 73.66,53.34 75.18,51.82 ARDUINO_DUE1.40
41  (via drill 0.35)
  Top 0.305: JP9.3 34.29,10.16 36.3,8.15 42.44,8.15 v46.99,12.7 | v85.09,36.83 85.09,34.29 82.53,31.73 81.28,31.73 79.65,30.1 79.65,27.78 80.01,27.43 v80.01,26.67
  Bottom 0.305: ARDUINO_DUE1.41 84.07,51.82 85.09,50.8 v85.09,36.83 | v80.01,26.67 77.47,24.13 58.42,24.13 v46.99,12.7
42  (via drill 0.35)
  Top 0.305: U1.11 58.03,53.73 v58.9,52.86
  Bottom 0.305: v58.9,52.86 62.48,49.28 ARDUINO_DUE1.42
43  (via drill 0.35)
  Top 0.305: ARDUINO_DUE1.43 90.42,49.28 91.44,48.26 91.44,24.13 v86.36,19.05
  Bottom 0.305: v86.36,19.05 86.36,7.62 85.09,6.35 U$5.J1.6
44  (via drill 0.35)
  Top 0.305: ARDUINO_DUE1.44 64.9,31.75 58.42,31.75 57.15,30.48 57.15,21.59 v52.07,16.51 | v45.72,10.16 43.18,7.62 34.8,7.62 31.75,10.67 27.43,10.67 22.86,15.24 R4.2
  Bottom 0.305: v52.07,16.51 v45.72,10.16
45  (via drill 0.35)
  Top 0.305: v85.09,24.13 90.17,29.21 90.17,44.45 87.88,46.74 ARDUINO_DUE1.45
  Bottom 0.305: U$5.J1.5 85.09,11.43 v85.09,24.13
46  (via drill 0.35)
  Top 0.305: U1.14 58.03,48.65 59.69,46.99 v60.96,46.99
  Bottom 0.305: v60.96,46.99 77.09,46.99 ARDUINO_DUE1.46
47  (via drill 0.35)
  Top 0.305: ARDUINO_DUE1.47 87.88,44.2 88.9,43.18 v88.9,29.21 | v87.63,21.59 U$5.J1.2
  Bottom 0.305: v88.9,29.21 88.9,22.86 v87.63,21.59
48  (via drill 0.35)
  Top 0.305: U1.13 57.38,48.02 v59.69,45.72
  Bottom 0.305: v59.69,45.72 71.12,45.72 75.18,41.66 ARDUINO_DUE1.48
49  (via drill 0.35)
  Top 0.305: v89.66,25.91 82.8,19.05 U$5.J1.1 | v87.63,40.64 83.44,40.64 ARDUINO_DUE1.49
  Bottom 0.305: v89.66,25.91 89.66,38.61 v87.63,40.64
50
  Bottom 0.305: JP4.5 57.15,39.37 57.15,34.29 59.69,31.75 69.85,31.75 77.22,39.12 ARDUINO_DUE1.50
51
  Top 0.305: U$6.J1.1 68.58,25.4 85.09,25.4 86.36,26.67 86.36,38.1 85.34,39.12 ARDUINO_DUE1.51
52  (via drill 0.35)
  Top 0.305: v24.13,16.51 v26.67,16.51 | v34.29,16.51 v36.83,16.51 | v57.15,31.75 58.42,33.02 v64.77,33.02 | v72.39,35.56 73.41,36.58 ARDUINO_DUE1.52
  Bottom 0.305: S1.1 19.09,7.66 21.59,10.16 21.59,15.24 22.86,16.51 v24.13,16.51 | v26.67,16.51 v34.29,16.51 | v36.83,16.51 43.18,16.51 44.76,18.09 44.76,18.18 45.32,18.74 45.41,18.74 50.8,24.13 55.88,24.13 57.15,25.4 v57.15,31.75 | v64.77,33.02 67.31,35.56 v72.39,35.56
53
  Bottom 0.305: ARDUINO_DUE1.53 84.07,36.58 85.22,35.43 85.22,26.8 80.01,21.59 66.04,21.59 64.77,20.32 64.77,19.05 U$6.J1.2
+3V3
  Top 0.508: JP4.1 64.53,41.67 U1.24 67.31,52.46 67.31,63.5 JP2.1
  Bottom 0.406: JP2.1 63.5,64.77 | JP1.1 60.96,67.31 63.5,64.77 | JP3.1 52.07,66.04 53.34,64.77 63.5,64.77 | 35.56,15.75 35.56,21.08
  Bottom 0.508: U$4.3V3 30.48,40.64 27.94,38.1 | 27.94,38.1 21.46,31.62 ARDUINO_DUE1.3V3 21.59,28.83 21.59,24.13 22.86,22.86 33.78,22.86 35.56,21.08 | 35.56,15.75 36.83,14.48 JP9.4 36.83,10.92 38.86,8.89 54.61,8.89 60.96,15.24 U$6.J1.3 66.04,15.24 69.85,11.43 69.85,3.81 71.12,2.54 77.47,2.54 78.74,3.81 78.74,12.7 80.01,13.97 U$5.J1.3 | 27.94,38.1 54.61,38.1 55.88,39.37 55.88,40.64 58.42,43.18 62.23,43.18 63.5,41.91 JP4.1
A0
  Top 0.406: U1.1 64.53,54.38 62.23,52.07 54.61,52.07 45.72,43.18 45.72,36.83 44.45,35.56 41.91,35.56 36.7,30.35 ARDUINO_DUE1.A0
A1  (via drill 0.46)
  Top 0.305: v44.45,41.91 41.91,44.45 v41.91,45.72
  Top 0.406: JP12.4 31.75,68.58 33.02,67.31 44.84,67.31 47.42,64.73 47.42,62.27 41.91,56.76 v41.91,53.34 | v50.8,40.64 50.32,40.64 44.68,35 43.89,35 39.37,30.48 39.37,29.08 ARDUINO_DUE1.A1
  Bottom 0.305: v41.91,53.34 v41.91,45.72
  Bottom 0.406: v50.8,40.64 49.53,40.64 48.26,41.91 v44.45,41.91
A2  (via drill 0.46)
  Top 0.406: v26.67,34.29 25.4,35.56 v25.4,38.1 | v13.97,53.34 v13.97,58.42 | v21.59,72.39 v24.13,72.39
  Bottom 0.406: ARDUINO_DUE1.A2 41.78,30.23 37.72,34.29 v26.67,34.29 | v25.4,38.1 22.86,35.56 16.51,35.56 13.97,38.1 v13.97,53.34 | v13.97,58.42 13.97,64.57 10.41,68.12 10.41,71.62 12.45,73.66 20.32,73.66 v21.59,72.39 | JP12.2 26.67,71.12 25.4,72.39 v24.13,72.39
A3  (via drill 0.46)
  Top 0.406: v43.18,39.37 39.37,35.56 v39.37,34.29
  Bottom 0.406: JP12.3 29.21,68.33 31.07,66.47 45.68,66.47 46.11,66.04 48.26,66.04 49.53,64.77 49.53,63.47 49.15,63.09 49.15,60.58 43.18,54.61 v43.18,39.37 | v39.37,34.29 41.91,34.29 44.32,31.88 ARDUINO_DUE1.A3
CH1  (via drill 0.46)
  Top 0.406: v55.88,66.04 58.42,63.5 58.42,59.91 59.34,58.99 U1.9
  Bottom 0.406: v55.88,66.04 54.61,66.04 53.19,67.46 53.19,69.04 52.07,70.16 JP3.2
CH2
  Top 0.406: U1.8 59.98,63.2 55.88,67.31 55.88,69.85 JP3.4
CH3
  Top 0.406: U1.7 60.63,66.36 58.42,68.58 58.42,69.85 JP3.6
CH4
  Top 0.406: U1.6 61.28,66.98 59.69,68.58 59.69,71.12 JP1.2
CH5
  Top 0.406: U1.5 61.94,65.75 64.77,68.58 64.77,71.12 JP1.4
CH6
  Top 0.406: U1.4 62.59,62.59 69.85,69.85 69.85,71.12 68.58,72.39 JP1.6
CH7  (via drill 0.46)
  Top 0.406: U1.3 63.23,60.7 64.77,62.23 v66.04,62.23
  Bottom 0.406: v66.04,62.23 67.31,63.5 69.85,63.5 JP2.4
CH8  (via drill 0.46)
  Top 0.406: U1.2 63.88,58.8 v64.77,59.69
  Bottom 0.406: v64.77,59.69 67.31,57.15 69.85,57.15 71.12,58.42 JP2.6
CH9  (via drill 0.46)
  Top 0.406: U1.23 63.88,52.45 v66.04,54.61
  Bottom 0.406: v66.04,54.61 72.39,54.61 73.66,55.88 73.66,63.5 72.39,64.77 JP2.2
CH10  (via drill 0.46)
  Top 0.406: U1.22 63.23,44.72 v63.5,44.45
  Bottom 0.406: v63.5,44.45 64.77,44.45 67.31,41.91 67.31,36.83 66.04,35.56 64.77,35.56 63.5,36.83 JP4.2
CH11  (via drill 0.46)
  Top 0.406: U1.21 62.59,46.08 v60.96,44.45 | v53.34,39.37 53.34,36.83 55.88,34.29 59.69,34.29 60.96,35.56 JP4.4
  Bottom 0.406: v60.96,44.45 54.61,44.45 53.34,43.18 v53.34,39.37
CH12
  Top 0.406: U1.20 61.94,46.7 59.69,44.45 57.15,44.45 54.61,41.91 54.61,38.1 55.88,36.83 57.15,36.83 JP4.6
E1
  Bottom 0.406: JP7.3 91.44,76.2 86.36,71.12 86.36,20.32 90.17,16.51 U$5.J2.2
E2  (via drill 0.46)
  Top 0.406: v90.17,19.05 90.17,16.51 v88.9,15.24
  Bottom 0.305: JP8.3 91.44,67.31 90.42,66.29
  Bottom 0.406: 90.42,66.29 90.42,19.3 v90.17,19.05 90.17,16.51 | v88.9,15.24 88.9,8.89 91.44,6.35 U$5.J2.6
E3  (via drill 0.46)
  Top 0.406: v67.31,11.43 67.31,16.51 68.58,17.78 U$6.J2.2
  Bottom 0.406: JP6.3 98.36,27.94 98.78,27.51 98.78,3.81 96.24,1.27 68.58,1.27 67.31,2.54 v67.31,11.43
GND  (via drill 0.35)
  Top 0.508: v29.46,21.84 30.48,22.86 v35.05,22.86
  Bottom 0.508: v29.46,21.84 29.72,21.59 30.48,21.59 | v35.05,22.86 33.27,24.64 30.99,24.64 29.08,26.54 ARDUINO_DUE1.GND_1
  pour Top (isolate 0.305): -0.25,100.33 100.33,100.33 100.33,-0.25 -0.25,-0.25
  pour Bottom (isolate 0.305): -0.25,100.08 -0.25,-0.51 100.33,-0.51 100.33,100.08
N$1
  Top 0.305: R1.2 LED1.C
N$2
  Top 0.305: LED2.C R2.2
N$3
  Top 0.305: LED3.C R3.2
  Top 0.406: LED3.C 22.86,95.25
N$4  (via drill 0.46)
  Top 0.406: JP10.2 27.43,2.54 26.67,3.3 T1.2 | v58.42,6.35 45.97,18.8 25.91,18.8 24.13,20.57 D1.A
  Bottom 0.406: v58.42,6.35 JP10.2
N$5
  Bottom 0.406: R4.1 22.86,5.08 23.62,4.32 28.19,4.32 29.21,5.33 T1.1
SCL  (via drill 0.35, 0.46)
  Top 0.305: v40.64,48.26 v48.26,48.26 | v66.04,63.5 67.51,64.97 67.51,65.21 68.14,65.84 68.38,65.84 72.26,69.72 ARDUINO_DUE1.21
  Top 0.406: U$4.SCL 35.56,31.75 34.29,30.48 34.29,26.67 v38.1,22.86 | v36.32,21.59 31.75,21.59 v30.48,20.32 | JP9.2 29.21,15.24 29.21,17.02 v29.97,17.78 45.72,17.78 v50.8,12.7 | SV1.3 45.47,7.11 v48.77,10.41
  Bottom 0.305: U$4.SCL 40.64,46.99 v40.64,48.26 | v48.26,48.26 53.34,48.26 62.23,57.15 62.23,60.96 64.77,63.5 v66.04,63.5
  Bottom 0.406: v38.1,22.86 36.83,21.59 v36.32,21.59 | v30.48,20.32 30.48,18.29 v29.97,17.78 | v48.77,10.41 50.04,11.68 50.29,11.68 50.8,12.19 v50.8,12.7
SDA  (via drill 0.35, 0.46)
  Top 0.406: ARDUINO_DUE1.20 67.44,74.93 52.07,74.93 48.26,71.12 48.26,58.42 33.02,43.18 U$4.SDA | v27.94,21.59 24.13,25.4 11.43,25.4 10.16,26.67 10.16,31.75 16.51,38.1 v20.32,38.1 | v27.69,17.78 27.69,14.22 JP9.1 | v32.77,8.13 31.24,9.65 v31.24,9.91
  Bottom 0.406: v20.32,38.1 20.32,43.18 22.86,45.72 32.26,45.72 33.02,44.96 U$4.SDA | v27.94,21.59 27.94,19.05 27.69,18.8 v27.69,17.78 | SV1.2 40.14,8.13 v32.77,8.13 | JP9.1 31.24,10.67 v31.24,9.91
T1
  Bottom 0.406: JP7.2 93.98,73.66 95.25,72.39 97.79,72.39 98.78,71.4 98.78,65.76 91.44,58.42 91.44,20.32 U$5.J2.1
T2  (via drill 0.46)
  Top 0.406: v92.71,62.23 92.71,24.13 86.36,17.78 86.36,10.16 v87.63,8.89
  Bottom 0.305: JP8.2 93.98,67.31 92.71,66.04 v92.71,62.23
  Bottom 0.406: v87.63,8.89 87.63,7.62 91.44,3.81 93.98,3.81 95,4.83 95,8.13 94.23,8.89 U$5.J2.5
T3  (via drill 0.46)
  Top 0.406: JP6.2 97.79,25.4 98.78,24.41 98.78,4.8 95.25,1.27 74.93,1.27 v71.12,5.08
  Bottom 0.406: v71.12,5.08 71.12,19.05 72.39,20.32 U$6.J2.1
VCC  (via drill 0.35, 0.46)
  Top 0.406: v57.15,10.16 55.88,10.16 v48.26,17.78 44.45,21.59 v40.64,21.59 | v36.83,9.14 40.39,9.14 41.91,10.67 JP9.6 43.18,13.97 v44.45,13.97 | D1.C 9.4,21.34 6.6,24.13 3.83,24.13 X1.1
  Bottom 0.406: JP10.1 60.96,8.89 59.69,10.16 v57.15,10.16 | X1.1 19.07,24.11 22.86,20.32 24.13,20.32 25.4,19.05 25.4,12.7 28.45,9.65 29.7,9.65 30.21,9.14 v36.83,9.14 | v44.45,13.97 44.45,16.51 45.72,17.78 v48.26,17.78
  Bottom 0.508: ARDUINO_DUE1.VIN 31.62,26.8 33.02,25.4 36.83,25.4 v40.64,21.59

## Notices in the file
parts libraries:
SparkFun-Switches: Licensing: Creative Commons ShareAlike 4.0 International - https://creativecommons.org/licenses/by-sa/4.0
diy-modules: Released under the Creative Commons Attribution 4.0 International License: http://creativecommons.org/licenses/by/4.0
